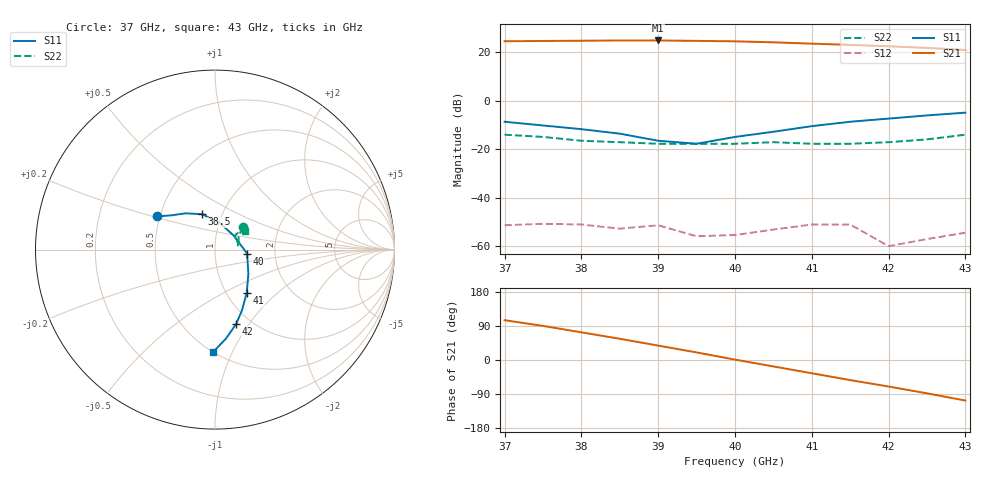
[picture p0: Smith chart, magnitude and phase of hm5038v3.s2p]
! HMMC-5038
! S-PARAMETERS at  Vdd = 3V;  Idd = 150mA. LAST UPDATED  02-24-97
# GHZ  S  MA  R 50
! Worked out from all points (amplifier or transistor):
!   13 points, 37 GHz to 43 GHz, reference 50 ohm
!   highest |S21| = 24.9 dB at 39 GHz (marker M1)
!   |S21| within 3 dB of that: start of sweep to 42.45 GHz
!   unconditionally stable (mu >= 1): start of sweep to end of sweep
!   at 38 GHz: K = 9.37, MAG = 25.2 dB, |S12| = -51.1 dB
!   at 40 GHz: K = 16.55, MAG = 24.8 dB, |S12| = -55.4 dB
!   at 43 GHz: K = 15.22, MAG = 22.9 dB, |S12| = -54.4 dB
!   S11 on the Smith chart (normalised r, x): 37 GHz: 0.49, +0.21; 38.5 GHz: 0.80, +0.33; 40 GHz: 1.43, -0.06; 41 GHz: 1.23, -0.66; 42 GHz: 0.86, -0.87; 43 GHz: 0.50, -0.85
37  0.37 150.0  16.99 105.0  0.0027 34.0  0.2 39.0
37.5  0.31 142.0  17.2 90.0  0.0029 14.0  0.18 36.0
38  0.26 129.0  17.4 73.0  0.0028 10.0  0.15 29.0
38.5  0.21 110.0  17.61 56.0  0.0023 7.0  0.14 20.0
39  0.15 79.0  17.63 38.0  0.0027 4.0  0.13 13.0
39.5  0.13 37.0  17.28 20.0  0.0016 -7.0  0.13 8.0
40  0.18 -7.0  16.9 1.0  0.0017 57.0  0.13 13.0
40.5  0.23 -36.0  16.14 -17.0  0.0022 27.0  0.14 16.0
41  0.3 -54.0  15.14 -35.0  0.0028 8.0  0.13 20.0
41.5  0.37 -66.0  14.29 -53.0  0.0028 -8.0  0.13 30.0
42  0.43 -74.0  13.36 -70.0  0.001 -37.0  0.14 36.0
42.5  0.5 -83.0  12.38 -88.0  0.0014 -12.0  0.16 36.0
43  0.57 -91.0  11.21 -107.0  0.0019 -39.0  0.2 32.0
